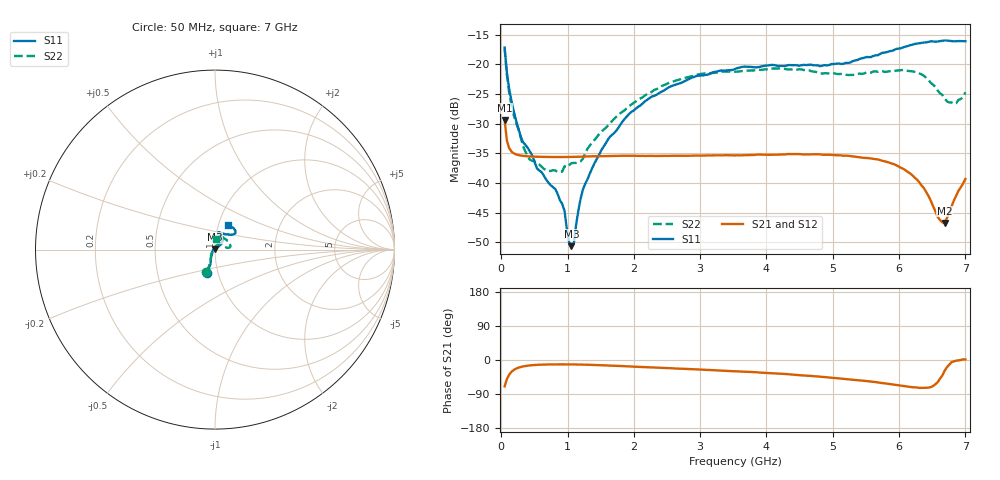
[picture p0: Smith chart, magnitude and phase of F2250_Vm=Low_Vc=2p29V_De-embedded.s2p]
! Integrated Device Technology
! Corporate Headquarters
! 6024 Silver Creek Valley Road
! San Jose, CA 95138  USA
! Phone:  1-408-284-8200
! Toll Free:  1-800-223-1366
! Webpage:  http://www.idt.com/
! Timing and RF Division
! 515 Groton Road, Suite 102
! Westford, MA 01886-6024
! Device:  F2250
! Description: Voltage Variable RF Attenuator
! Frequency:  50.0 -  6000.00 MHz
! Package:  3x3 mm Thin QFN Plastic Package: 16 pin
! Ports:  2 RF, 3 DC
!  Pin  1  = GND
!  Pin  2  = NC
!  Pin  3  = RF1  = Port 1
!  Pin  4  = NC
!  Pin  5  = GND
!  Pin  6  = GND
!  Pin  7  = GND
!  Pin  8  = GND
!  Pin  9  = NC
!  Pin 10  = RF2  = Port 2
!  Pin 11  = NC
!  Pin 12  = GND
!  Pin 13  = GND
!  Pin 14  = VCNTRL
!  Pin 15  = VDD
!  Pin 16  = VMODE
! Vcntrl:  2.290 Volts
! Vmode:  +0.000 Volts
! Vdd:  +3.30  Volts
! Current:  1.177 mA
! Data:  The device was measured on a the F2250 evaluation board which has
!  individual transmission lines to the RF pins.  Data was collected
!  using a calibrated network analyzer.  The evaluation board was
!  de-embedded using a TRL calibration technique.
!  The reference plane is the edge of the package pin.
! Misc:  SN 10
!  Action Tracker AT0258
! Date Measured:  2014-11-26
! Date:  2015-10-15  MJV
! Note:
!  Integrated Device Technology supplies this data as a sample of measured
!  data at the package pin for this product.  Your particular data for this
!  product may vary.
!  Data was taken at 25 degrees C.
!  Integrated Device Technology reserves the right to change this data at anytime.
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# GHz S dB R 50
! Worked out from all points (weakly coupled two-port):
!   201 points, 50 MHz to 7 GHz, reference 50 ohm
!   highest |S21| = -29.40 dB at 50 MHz (marker M1); lowest = -46.8 dB at 6.687 GHz (marker M2)
!   lowest |S11| = -50.7 dB at 1.058 GHz (marker M3), VSWR 1.01, Z = 49.8 + j0.244 ohm
!   |S11| at or under -10 dB: start of sweep to end of sweep
!   |S22| runs from -38.2 to -17.3 dB; largest |S21 - S12| = 6.4e-05
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0.05  -17.18 -108.6  -29.40 -69.7  -29.40 -69.7  -17.32 -110.8
0.08475  -21.45 -107.5  -32.89 -50.2  -32.89 -50.2  -21.83 -109.6
0.15425  -26.23 -116.6  -34.73 -31.0  -34.72 -31.1  -26.96 -121.4
0.29325  -32.20 -127.9  -35.40 -18.4  -35.39 -18.4  -32.38 -135.9
0.3975  -34.09 -141.8  -35.52 -15.0  -35.52 -15.0  -35.55 -159.2
0.91875  -43.54 158.2  -35.65 -11.5  -35.64 -11.5  -38.11 130.9
0.9535  -44.71 169.8  -35.65 -11.6  -35.65 -11.5  -37.19 128.7
1.023  -50.02 143.9  -35.64 -11.6  -35.64 -11.6  -37.02 112.7
1.05775  -50.68 123.1  -35.63 -11.6  -35.63 -11.6  -36.67 107.5
1.0925  -50.33 89.8  -35.62 -11.7  -35.62 -11.7  -36.65 102.6
1.162  -44.69 56.6  -35.60 -11.9  -35.60 -11.9  -36.47 91.9
1.2315  -41.11 44.4  -35.57 -12.1  -35.57 -12.1  -35.91 82.4
1.61375  -32.61 40.9  -35.49 -14.5  -35.49 -14.5  -30.30 63.6
1.9265  -28.40 41.3  -35.43 -16.9  -35.43 -16.9  -27.08 55.3
2.37825  -24.88 47.4  -35.45 -20.3  -35.44 -20.3  -24.01 55.9
3.525  -20.80 72.5  -35.37 -29.6  -35.38 -29.6  -21.27 74.3
4.7065  -20.17 72.3  -35.18 -42.6  -35.17 -42.6  -21.24 72.0
5.85325  -17.81 40.5  -36.60 -63.3  -36.60 -63.3  -21.19 22.5
6.27025  -16.51 40.1  -39.45 -72.6  -39.46 -72.7  -21.40 9.2
6.68725  -15.99 48.8  -46.77 -28.3  -46.75 -28.1  -25.74 28.0
6.861  -16.13 55.1  -42.17 -1.8  -42.12 -1.7  -26.59 58.0
7  -16.12 63.2  -39.35 1.5  -39.30 1.4  -24.72 83.4
